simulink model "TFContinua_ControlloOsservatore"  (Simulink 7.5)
settings: Solver=ode45  StartTime=0.0  StopTime=10.0  FixedStep=Ts  RelTol=1e-3
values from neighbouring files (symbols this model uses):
  As1 = 1    [TSC160720ProvaMatlab.m]
  As2 = 2    [TSC160720ProvaMatlab.m]
  Kff = -inv(Cz*inv(Az-Bz*K-eye(n))*Bz)    [TSC160720ProvaMatlab.m]
  L = -acker(Az',Cz',[0 0 0])'    [TSC160720ProvaMatlab.m]
  Ts = time(2)-time(1)    [TSC160720ProvaMatlab.m]
  ts1 = 0    [TSC160720ProvaMatlab.m]
  ts2 = 5    [TSC160720ProvaMatlab.m]
undefined symbols (not defined in the file or in its folder): Az, Bz, Cz, K
libraries: cstblocks x1

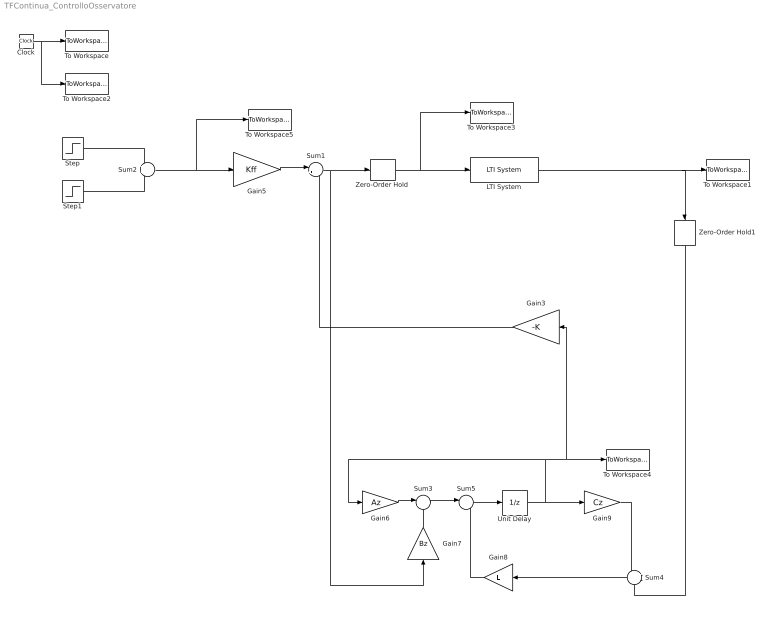
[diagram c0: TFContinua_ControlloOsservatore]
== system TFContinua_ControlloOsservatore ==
  Clock : Clock
  Gain3 : Gain  Gain=-K  Multiplication=Matrix(K*u)
  Gain5 : Gain  Gain=Kff  Multiplication=Matrix(K*u)
  Gain6 : Gain  Gain=Az  Multiplication=Matrix(K*u)
  Gain7 : Gain  Gain=Bz  Multiplication=Matrix(K*u)
  Gain8 : Gain  Gain=L  Multiplication=Matrix(K*u)
  Gain9 : Gain  Gain=Cz  Multiplication=Matrix(K*u)
  LTI System : cstblocks/LTI System  SystemSampleTime=-1  sys=G  IC=[]
  Step : Step  Time=ts1  After=As1  SampleTime=0
  Step1 : Step  Time=ts2  After=As2  SampleTime=0
  Sum1 : Sum  Inputs=|++
  Sum2 : Sum
  Sum3 : Sum  Inputs=|++
  Sum4 : Sum  Inputs=+-
  Sum5 : Sum  Inputs=|++
  To Workspace : ToWorkspace  VariableName=time  SampleTime=-1  SaveFormat=Array
  To Workspace1 : ToWorkspace  VariableName=y  SampleTime=-1  SaveFormat=Array
  To Workspace2 : ToWorkspace  VariableName=timed  SampleTime=Ts  SaveFormat=Array
  To Workspace3 : ToWorkspace  VariableName=u  SampleTime=-1  SaveFormat=Array
  To Workspace4 : ToWorkspace  VariableName=Xs  SampleTime=-1  SaveFormat=Array
  To Workspace5 : ToWorkspace  VariableName=yref  SampleTime=-1  SaveFormat=Array
  Unit Delay : UnitDelay  SampleTime=Ts
  Zero-Order Hold : ZeroOrderHold  SampleTime=Ts
  Zero-Order Hold1 : ZeroOrderHold  SampleTime=Ts
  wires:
  LTI System/1 -> To Workspace1/1, Zero-Order Hold1/1
  Clock/1 -> To Workspace2/1, To Workspace/1
  Gain6/1 -> Sum3/1
  Unit Delay/1 -> Gain9/1, Gain6/1, Gain3/1, To Workspace4/1
  Gain7/1 -> Sum3/2
  Sum4/1 -> Gain8/1
  Gain9/1 -> Sum4/1
  Gain8/1 -> Sum5/2
  Sum3/1 -> Sum5/1
  Sum5/1 -> Unit Delay/1
  Gain5/1 -> Sum1/1
  Sum1/1 -> Zero-Order Hold/1, Gain7/1
  Gain3/1 -> Sum1/2
  Step/1 -> Sum2/1
  Step1/1 -> Sum2/2
  Sum2/1 -> To Workspace5/1, Gain5/1
  Zero-Order Hold/1 -> To Workspace3/1, LTI System/1
  Zero-Order Hold1/1 -> Sum4/2
